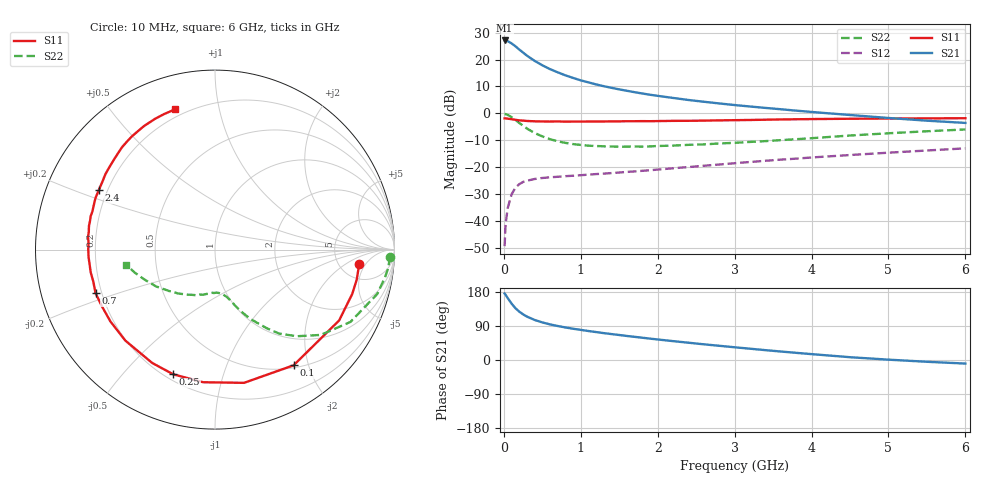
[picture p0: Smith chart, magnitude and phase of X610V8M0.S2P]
! SIEMENS Small Signal Semiconductors
! BFP193W
! Si NPN RF Bipolar Junction Transistor in SOT343
! VCE = 10 V  IC = 8 mA
! Common Emitter S-Parameters:  April 1994
# GHz  S  MA  R  50
!  f  S11  S21  S12  S22
! GHz  MAG  ANG  MAG  ANG  MAG  ANG  MAG  ANG
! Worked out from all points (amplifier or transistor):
!   40 points, 10 MHz to 6 GHz, reference 50 ohm
!   highest |S21| = 27.1 dB at 10 MHz (marker M1)
!   |S21| within 3 dB of that: start of sweep to 184.9 MHz
!   unconditionally stable (mu >= 1): 1.501 GHz to 4.584 GHz
!   at 200 MHz: K = 0.19, MSG = 25.0 dB, |S12| = -26.3 dB
!   at 1.5 GHz: K = 1.00, MSG = 15.5 dB, |S12| = -22.0 dB
!   at 6 GHz: K = 0.92, MSG = 4.7 dB, |S12| = -13.0 dB
!   S11 on the Smith chart (normalised r, x): 10 MHz: 7.72, -3.56; 100 MHz: 0.54, -1.76; 250 MHz: 0.23, -0.69; 700 MHz: 0.18, -0.17; 2.4 GHz: 0.17, +0.24; 6 GHz: 0.16, +0.74
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0.01  0.8075 -5.7  22.65 175.5  0.0034 80.7  0.9765 -2.3
0.02  0.8072 -11.9  22.62 173.1  0.0074 79.1  0.9698 -6.3
0.03  0.8036 -17.9  22.52 169.9  0.0105 79.3  0.9596 -9.3
0.05  0.7964 -29.7  21.97 163.4  0.0173 74.6  0.9373 -15.3
0.1  0.7793 -55.8  20 149.0  0.0311 62.7  0.8555 -28.1
0.15  0.7598 -77.7  17.68 136.8  0.0415 52.9  0.7571 -38.9
0.2  0.7419 -95.1  15.37 127.7  0.0482 46.0  0.6644 -46.6
0.25  0.7327 -108.5  13.5 120.5  0.0531 41.0  0.5892 -52.6
0.3  0.7221 -119.0  11.83 114.6  0.0559 37.5  0.5221 -56.8
0.4  0.7118 -134.6  9.468 105.7  0.0603 32.7  0.4321 -63.1
0.5  0.707 -145.5  7.825 99.2  0.0629 30.3  0.3727 -67.2
0.6  0.7049 -153.5  6.643 94.0  0.0648 29.1  0.3312 -70.3
0.7  0.7083 -160.0  5.792 89.7  0.0663 28.9  0.3022 -72.5
0.9  0.704 -169.6  4.553 82.5  0.0693 29.3  0.2684 -76.6
1.1  0.7057 -176.6  3.764 76.5  0.0727 30.6  0.2508 -80.2
1.6  0.7144 169.4  2.628 63.4  0.0816 34.9  0.2403 -89.2
2.2  0.7254 156.6  1.935 49.8  0.0954 39.2  0.2517 -100.9
2.4  0.7274 152.7  1.772 45.6  0.1004 40.2  0.26 -104.7
3.2  0.7533 138.6  1.342 29.8  0.1247 42.1  0.2944 -121.4
4.5  0.7941 119.8  0.932 7.4  0.1681 39.8  0.3874 -148.1
5.5  0.8067 110.5  0.731 -4.7  0.2041 36.0  0.465 -164.0
6  0.8122 106.0  0.664 -9.4  0.2238 34.0  0.5021 -170.3
